[IBIS Ver]   4.0
[Comment Char] |_char
[File name]   pse84_bga220.ibs
[File Rev] 1.2
[Date] 10/27/2023
[Source] Infineon Technologies IBIS team
[Notes]
|Rev. 1.0 - Initial model 12/8/2021
|Rev. 1.1 - Update with RLC 8/17/2023
|Rev. 1.2 - Included pins for MIPI-DPHY DSI and USB 10/23/2023
|Supports 1.8 V IO Interface and 3.3 V RF Switch Control Interface.
|The temperature range is -40 to 125C.
|This model was syntax checked with Hyperlynx 4.2 visual IBIS
|editor and ibischk7_64 IBIS checker.
|There were 0 syntax errors.
[Disclaimer]   The model given below represents a 220-pin package.
[Copyright]   (C) COPYRIGHT 2023, Infineon Technologies AG.
[Component] PSOCE84
[Manufacturer] Infineon Technologies AG
| Package model BGA220 was extracted from simulation tool.
[Package]
|   typ   min   max
R_pkg   0.20796   0.07347   0.41266
L_pkg   2.2356n   0.87131n   4.135n
C_pkg   0.96052p   0.4552p   1.843p
[Pin]   Signal_name   model_name   R_pin   L_pin   C_pin
|A4   DSI_CLK_N_PAD   PAD   0.20054 2.35E-09 5.53E-13
|A5   DSI_CLK_P_PAD   PAD   0.16186 1.88E-09 4.79E-13
|B4   DSI_DATA0_N_PAD PAD   0.17864 1.75E-09 9.29E-13
|B3   DSI_DATA0_P_PAD PAD   0.2296  2.45E-09 8.54E-13
|A3   DSI_DATA1_N_PAD PAD   0.1872  2.24E-09 5.28E-13
|A2   DSI_DATA1_P_PAD PAD   0.23123 2.69E-09 6.88E-13
|J6   DSI_REXT_PAD   0.36792 3.61E-09 1.32E-12
K5   P0_0_PAD   Mpad 0.22656 2.30E-09 1.44E-12
C4   P0_1_PAD   Mpad 0.22018 2.42E-09 1.02E-12
B15   P10_0_PAD   1p8_ioi2c_wbso_h   0.21635 2.63E-09  6.76E-13
A13   P10_1_PAD   1p8_ioi2c_wbso_h   0.18836 2.05E-09  8.54E-13
C15   P10_2_PAD   1p8_ioi2c_wbso_h   0.2   2.52E-09  4.58E-13
A14   P10_3_PAD   1p8_ioi2c_wbso_h   0.2025  2.35E-09  7.28E-13
D14   P10_4_PAD   1p8_ioi2c_wbso_h   0.17929 2.22E-09  5.12E-13
B14   P10_5_PAD   1p8_ioi2c_wbso_h   0.18293 2.02E-09  8.32E-13
D15   P10_6_PAD   1p8_ioi2c_wbso_h   0.18633 2.26E-09  4.55E-13
C14   P10_7_PAD   1p8_ioi2c_wbso_h   0.16378 1.74E-09  8.10E-13
E14   P11_0_PAD   1p8_ovt_wbso_h  0.15753 1.75E-09   5.94E-13
E11   P11_1_PAD   1p8_ovt_wbso_h  0.13177 1.35E-09   1.04E-12
E15   P11_2_PAD   1p8_ovt_wbso_h  0.18244 2.22E-09   5.01E-13
E10   P11_3_PAD   1p8_ovt_wbso_h  0.16649 1.81E-09   9.34E-13
F14   P11_4_PAD   1p8_ovt_wbso_h  0.16571 1.97E-09   5.83E-13
F9   P11_5_PAD   1p8_ovt_wbso_h  0.16904 1.76E-09   1.03E-12
F13   P11_6_PAD   1p8_ovt_wbso_h  0.16654 1.72E-09   6.89E-13
F10   P11_7_PAD   1p8_ovt_wbso_h  0.14172 1.43E-09   9.11E-13
H5   P12_0_PAD   1p8_ioi2c_wbso_h   0.22824 2.31E-09   1.72E-12
D5   P12_1_PAD   1p8_ioi2c_wbso_h   0.3004  3.07E-09   1.08E-12
G5   P12_2_PAD   1p8_ioi2c_wbso_h   0.21503 2.22E-09   1.67E-12
E5   P12_3_PAD   1p8_ioi2c_wbso_h   0.3353  3.50E-09   1.22E-12
F4   P12_4_PAD   1p8_ioi2c_wbso_h   0.21904 2.27E-09   1.70E-12
F5   P12_5_PAD   1p8_ioi2c_wbso_h   0.35086 3.67E-09   1.26E-12
G8   P13_0_PAD   1p8_gpib_3swbso_h   0.17914 1.89E-09   1.14E-12
G9   P13_1_PAD   1p8_ioi2c_wbso_h   0.19087 1.96E-09   1.12E-12
G10   P13_2_PAD   1p8_ioi2c_wbso_h   0.16512 1.71E-09   1.02E-12
F15   P13_3_PAD   1p8_ioi2c_wbso_h   0.17042 1.84E-09   6.52E-13
G11   P13_4_PAD   1p8_ioi2c_wbso_h   0.11221 1.14E-09   9.78E-13
G14   P13_5_PAD   1p8_gpib_3swbso_h   0.17144 1.82E-09   5.45E-13
H11   P13_6_PAD   1p8_ioi2c_wbso_h   0.13435 1.39E-09   1.17E-12
H15   P13_7_PAD   1p8_ioi2c_wbso_h   0.1915  2.03E-09   5.03E-13
H10   P14_0_PAD   1p8_gpib_3swbso_h   0.16351 1.69E-09   1.38E-12
H13   P14_1_PAD   1p8_ioi2c_wbso_h   0.16226 1.59E-09   6.35E-13
H9   P14_2_PAD   1p8_ioi2c_wbso_h   0.18536 1.94E-09   1.41E-12
K15   P14_3_PAD   1p8_ioi2c_wbso_h   0.21748 2.73E-09   6.39E-13
J9   P14_4_PAD   1p8_ioi2c_wbso_h   0.17465 1.83E-09   1.32E-12
J15   P14_5_PAD   1p8_gpib_3swbso_h   0.17014 2.04E-09   5.24E-13
J10   P14_6_PAD   1p8_ioi2c_wbso_h   0.165   1.67E-09   1.02E-12
J14   P14_7_PAD   1p8_ioi2c_wbso_h   0.15607 1.59E-09   6.84E-13
L15   P15_0_PAD   1p8_ioi2c_wbso_h   0.17878 1.99E-09   6.08E-13
K13   P15_1_PAD   1p8_ioi2c_wbso_h   0.09136 9.76E-10   7.13E-13
M15   P15_2_PAD   1p8_ioi2c_wbso_h   0.21222 2.46E-09   6.00E-13
K9   P15_3_PAD   1p8_ioi2c_wbso_h   0.18524 1.95E-09   1.08E-12
N15   P15_4_PAD   1p8_ioi2c_wbso_h   0.21678 2.49E-09   7.87E-13
K10   P15_5_PAD   1p8_ioi2c_wbso_h   0.14996 1.62E-09   1.01E-12
P15   P15_6_PAD   1p8_ioi2c_wbso_h   0.26151 3.03E-09   7.66E-13
K11   P15_7_PAD   1p8_ioi2c_wbso_h   0.13152 1.43E-09   1.09E-12
M11   P16_0_PAD   3p3_gpio_wbso_v 0.15372 1.78E-09   8.07E-13
R13   P16_1_PAD   3p3_gpio_wbso_v 0.20685 2.25E-09   9.30E-13
N11   P16_2_PAD   3p3_gpio_wbso_v 0.18636 2.08E-09   8.28E-13
L11   P16_3_PAD   3p3_gpio_wbso_v 0.083686   9.67E-10   8.68E-13
P11   P16_4_PAD   3p3_gpio_wbso_v 0.21434 2.37E-09   8.02E-13
L10   P16_5_PAD   3p3_gpio_wbso_v 0.07347 8.73E-10   1.03E-12
R11   P16_6_PAD   3p3_gpio_wbso_v 0.22038 2.44E-09   7.88E-13
M10   P16_7_PAD   3p3_gpio_wbso_v 0.084206   9.06E-10   7.71E-13
M9   P17_0_PAD   3p3_gpio_wbso_v 0.15721 1.77E-09   8.06E-13
R9   P17_1_PAD   3p3_gpio_wbso_v 0.18702 1.89E-09   8.89E-13
R8   P17_2_PAD   3p3_gpio_wbso_v 0.22427 2.51E-09   8.66E-13
P9   P17_3_PAD   3p3_gpio_wbso_v 0.15414 1.64E-09   9.02E-13
P8   P17_4_PAD   3p3_gpio_wbso_v 0.19733 2.23E-09   8.36E-13
N9   P17_5_PAD   3p3_gpio_wbso_v 0.12454 1.32E-09   9.02E-13
N8   P17_6_PAD   3p3_gpio_wbso_v 0.18534 2.07E-09   8.23E-13
L9   P17_7_PAD   3p3_gpio_wbso_v 0.088819   9.54E-10   8.43E-13
G7   P18_0_PAD   1p8_gpib_3swbso_v   0.37774 3.96E-09   1.23E-12
H8   P18_1_PAD   1p8_gpib_3swbso_v   0.23204 2.41E-09   1.75E-12
B6   P19_0_PAD   1p8_gpib_3swbso_v   0.19164 2.27E-09   6.28E-13
F8   P19_1_PAD   1p8_gpib_3swbso_v   0.1648  1.77E-09   1.31E-12
K4   P2_0_PAD   Mpad   0.19132 1.92E-09   1.10E-12
P14   P20_0_PAD   1p8_ioi2c_wbso_h   0.22796 2.31E-09   1.03E-12
M12   P20_1_PAD   1p8_ioi2c_wbso_h   0.16258 1.85E-09   8.37E-13
R15   P20_2_PAD   1p8_ioi2c_wbso_h   0.24673 2.75E-09   9.68E-13
N12   P20_3_PAD   1p8_ioi2c_wbso_h   0.18993 2.15E-09   8.18E-13
R14   P20_4_PAD   1p8_ioi2c_wbso_h   0.24853 2.76E-09   9.15E-13
P12   P20_5_PAD   1p8_ioi2c_wbso_h   0.22155 2.48E-09   8.21E-13
P13   P20_6_PAD   1p8_ioi2c_wbso_h   0.17567 1.91E-09   9.23E-13
R12   P20_7_PAD   1p8_ioi2c_wbso_h   0.22524 2.55E-09   8.09E-13
J5   P21_0_PAD   1p8_ioi2c_wbso_h   0.23138 2.31E-09   1.55E-12
E4   P21_1_PAD   1p8_ioi2c_wbso_h   0.30704 3.17E-09   1.20E-12
K7   P21_2_PAD   1p8_ioi2c_wbso_h   0.27883 2.80E-09   1.64E-12
D4   P21_3_PAD   1p8_ioi2c_wbso_h   0.29341 3.06E-09   1.12E-12
K6   P21_4_PAD   1p8_ioi2c_wbso_h   0.24937 2.54E-09   1.56E-12
C5   P21_5_PAD   1p8_ioi2c_wbso_h   0.26732 2.84E-09   1.20E-12
L7   P21_6_PAD   1p8_ioi2c_wbso_h   0.28784 2.87E-09   1.52E-12
C3   P21_7_PAD   1p8_ioi2c_wbso_h   0.19023 2.11E-09   8.90E-13
M4   P3_0_PAD   1p8_ioi3c_3swbso_h   0.27521 2.73E-09   1.22E-12
L6   P3_1_PAD   1p8_ioi3c_3swbso_h   0.17463 1.82E-09   1.35E-12
J4   P5_0_PAD   Mpad   0.14852 1.49E-09   1.56E-12
M6   P6_0_PAD   1p8_ioi2c_wbso_h   0.15505 1.69E-09   8.65E-13
N6   P6_1_PAD   1p8_ioi2c_wbso_h   0.18486 2.04E-09   8.54E-13
P6   P6_2_PAD   1p8_ioi2c_wbso_h   0.21336 2.35E-09   7.99E-13
R6   P6_3_PAD   1p8_ioi2c_wbso_h   0.21761 2.42E-09   7.36E-13
R5   P6_4_PAD   1p8_ioi2c_wbso_h   0.22859 2.43E-09   1.00E-12
R2   P6_5_PAD   1p8_ioi2c_wbso_h   0.29623 3.21E-09   8.98E-13
P5   P6_6_PAD   1p8_ioi2c_wbso_h   0.20466 2.15E-09   1.01E-12
P2   P6_7_PAD   1p8_ioi2c_wbso_h   0.29712 2.98E-09   9.31E-13
P3   P7_0_PAD   1p8_ioi2c_wbso_h   0.27636 2.60E-09   1.03E-12
N5   P7_1_PAD   1p8_ioi2c_wbso_h   0.21064 2.19E-09   1.09E-12
R4   P7_2_PAD   1p8_ioi2c_wbso_h   0.30429 3.15E-09   1.15E-12
M5   P7_3_PAD   1p8_ioi2c_wbso_h   0.19338 2.05E-09   1.23E-12
P4   P7_4_PAD   1p8_ioi2c_wbso_h   0.2891  2.98E-09   1.13E-12
L4   P7_5_PAD   1p8_ioi2c_wbso_h   0.1324  1.41E-09   1.15E-12
N4   P7_6_PAD   1p8_ioi2c_wbso_h   0.29217 2.90E-09   1.15E-12
L5   P7_7_PAD   1p8_ioi2c_wbso_h   0.14611 1.56E-09   1.23E-12
H7   P8_0_PAD   1p8_ioi2c_wbso_h   0.39168 3.83E-09   1.31E-12
J8   P8_1_PAD   1p8_ioi2c_wbso_h   0.25811 2.68E-09   1.84E-12
J7   P8_2_PAD   1p8_ioi2c_wbso_h   0.41266 4.14E-09   1.43E-12
K8   P8_3_PAD   1p8_ioi2c_wbso_h   0.2804  2.80E-09   1.78E-12
F6   P8_4_PAD   1p8_ioi2c_wbso_h   0.27559 2.68E-09   1.04E-12
E7   P8_5_PAD   1p8_ioi2c_wbso_h   0.11114 1.15E-09   1.42E-12
G6   P8_6_PAD   1p8_ioi2c_wbso_h   0.29663 3.02E-09   1.19E-12
H6   P8_7_PAD   1p8_ioi2c_wbso_h   0.32423 3.31E-09   1.25E-12
L14   P9_0_PAD   1p8_ioi2c_wbso_h   0.11336 1.28E-09   6.46E-13
M13   P9_1_PAD   1p8_ioi2c_wbso_h   0.16723 1.93E-09   8.46E-13
M14   P9_2_PAD   1p8_ioi2c_wbso_h   0.15087 1.58E-09   8.83E-13
N13   P9_3_PAD   1p8_ioi2c_wbso_h   0.19382 2.18E-09   8.16E-13
L1   SMIF0_CLK_N_PAD Mpad_0   0.23622 2.67E-09   6.87E-13
M1   SMIF0_CLK_P_PAD Mpad_1   0.25153 2.76E-09   7.75E-13
N2   SMIF0_DATA0_PAD Mpad   0.29527 3.06E-09   1.12E-12
P1   SMIF0_DATA1_PAD Mpad   0.31791 3.40E-09   1.18E-12
N1   SMIF0_DATA2_PAD Mpad   0.31365 3.42E-09   9.23E-13
M2   SMIF0_DATA3_PAD Mpad   0.27296 2.87E-09   1.01E-12
L2   SMIF0_DATA4_PAD Mpad   0.25293 2.77E-09   9.73E-13
K2   SMIF0_DATA5_PAD Mpad   0.26485 2.86E-09   1.06E-12
K1   SMIF0_DATA6_PAD Mpad   0.26877 2.90E-09   8.60E-13
J2   SMIF0_DATA7_PAD Mpad   0.25994 2.81E-09   8.99E-13
J1   SMIF0_RWDS_PAD  Mpad   0.20375 2.49E-09   6.18E-13
F1   SMIF1_CLK_N_PAD Mpad_0   0.1842  2.21E-09   5.56E-13
E1   SMIF1_CLK_P_PAD Mpad_1   0.18934 2.20E-09   5.44E-13
C2   SMIF1_DATA0_PAD Mpad   0.18423 2.07E-09   7.99E-13
C1   SMIF1_DATA1_PAD Mpad   0.20375 2.29E-09   6.75E-13
D2   SMIF1_DATA2_PAD Mpad   0.18525 2.19E-09   6.35E-13
D1   SMIF1_DATA3_PAD Mpad   0.19093 2.32E-09   6.19E-13
F2   SMIF1_DATA4_PAD Mpad   0.19204 2.11E-09   7.77E-13
E2   SMIF1_DATA5_PAD Mpad   0.16192 1.78E-09   1.00E-12
G2   SMIF1_DATA6_PAD Mpad   0.1669  1.84E-09   7.17E-13
H2   SMIF1_DATA7_PAD Mpad   0.19427 2.18E-09   7.47E-13
H1   SMIF1_RWDS_PAD  Mpad   0.19851 2.24E-09   6.91E-13
|P7   USB_DM_PAD   PAD  0.20896 1.96E-09   8.83E-13
|N7   USB_DP_PAD   PAD  0.18134 1.68E-09   8.75E-13
H4   VCCD_0_PAD   POWER
F11   VCCD_1_PAD   POWER
E9   VCCD_2_PAD   POWER
M8   VCCD_3_PAD   POWER
B1   VCCD_4_PAD   POWER
B7   VCCD_ANA_PAD   POWER
B12   VCCI_SR_0_PAD   POWER
B13   VCCI_SR1P8_0_PAD   POWER
B9   VCCIRETLDO_PAD  POWER
C9   VCCRET_PAD   POWER
A8   VCCSRAM_PAD   POWER
F12   VCCSRAMI_0_PAD  POWER
K3   VCCSRAMI_1_PAD  POWER
M7   VDD33_USB_PAD   POWER
H14   VDDA_CTB_PAD   POWER
J12   VDDA_PAD   POWER
J11   VDDA_SAR_PAD   POWER
D10   VDDBAT_0_PAD   POWER
B11   VDDBAT_SR_PAD   POWER
G4   VDDD_DLL_PAD   POWER
A7   VDDD_PAD   POWER
B10   VDDD_SR_PAD   POWER
C12   VDDD_SR1P8_PAD  POWER
B8   VDDDLDO_PAD   POWER
R3   VDDIO_0_PAD   POWER
E6   VDDIO_1_PAD   POWER
R10   VDDIO_1P8_3P3_PAD   POWER
N14   VDDIO_2_PAD   POWER
E13   VDDIO_3_PAD   POWER
B2   VDDIO_4_PAD   POWER
G12   VDDIO_A_PAD   POWER
L12   VDDIO_A_Q_PAD   POWER
A6   VDDIO_CO_PAD   POWER
M3   VDDIO_SMIF0_0_PAD   POWER
J3   VDDIO_SMIF0_1_PAD   POWER
E3   VDDIO_SMIF1_0_PAD   POWER
G3   VDDIO_SMIF1_1_PAD   POWER
A12   VDDLX_SR_PAD   POWER
C13   VDDLX_SR1P8_PAD POWER
P10   VDDP_PAD   POWER
F7   VDDPUMP_RRAM_PAD   POWER
A11   VDDQ_0_PAD   POWER
A10   VDDQ_SR_PAD   POWER
A9   VDDQ_SR1P8_PAD  POWER
C6   VP_DSI_PAD   POWER
D6   VPH_P_DSI_PAD   POWER
C7   VPL_P_DSI_PAD   POWER
K14   VREF_PAD   POWER
C11   VSS_SR_PAD   GND
D12   VSS_SR1P8_PAD   GND
R7   VSS_USB_PAD   GND
G13   VSSA   GND
H12   VSSA   GND
J13   VSSA   GND
K12   VSSA   GND
L13   VSSA   GND
B5   VSSD   GND
D11   VSSD   GND
D13   VSSD   GND
D3   VSSD   GND
D7   VSSD   GND
E12   VSSD   GND
E8   VSSD   GND
F3   VSSD   GND
H3   VSSD   GND
L3   VSSD   GND
L8   VSSD   GND
N10   VSSD   GND
N3   VSSD   GND
C10   VSSQ_PAD   GND
C8   VSSQ_PAD   GND
D9   VSSQ_PAD   GND
D8   XRES_PAD   1p8_xres_3swbso 0.088991   9.56E-10   7.58E-13
[Diff_pin]   inv_pin   vdiff   tdelay_typ   tdelay_min   tdelay_max
E1   F1   0.2   -40.2244p   NA   NA
M1   L1   0.2   -40.2244p   NA   NA
|   MODEL SELECTOR
[Model Selector] 1p8_ioi2c_wbso_h
| Model Description
ioi2c_drive000_slew0   obuf mode with drive_sel=000 and slew_sel=0
ioi2c_drive000_slew1   obuf mode with drive_sel=000 and slew_sel=1
ioi2c_drive100_slew0   obuf mode with drive_sel=100 and slew_sel=0
ioi2c_drive100_slew1   obuf mode with drive_sel=100 and slew_sel=1
ioi2c_drive010_slew0   obuf mode with drive_sel=010 and slew_sel=0
ioi2c_drive010_slew1   obuf mode with drive_sel=010 and slew_sel=1
ioi2c_drive110_slew0   obuf mode with drive_sel=110 and slew_sel=0
ioi2c_drive110_slew1   obuf mode with drive_sel=110 and slew_sel=1
ioi2c_drive001_slew0   obuf mode with drive_sel=001 and slew_sel=0
ioi2c_drive001_slew1   obuf mode with drive_sel=001 and slew_sel=1
ioi2c_drive101_slew0   obuf mode with drive_sel=101 and slew_sel=0
ioi2c_drive101_slew1   obuf mode with drive_sel=101 and slew_sel=1
ioi2c_drive011_slew0   obuf mode with drive_sel=011 and slew_sel=0
ioi2c_drive011_slew1   obuf mode with drive_sel=011 and slew_sel=1
ioi2c_drive111_slew0   obuf mode with drive_sel=111 and slew_sel=0
ioi2c_drive111_slew1   obuf mode with drive_sel=111 and slew_sel=1
ioi2c_drive000_slow1   obuf mode with drive_sel=000 and slow=1
ioi2c_drive100_slow1   obuf mode with drive_sel=100 and slow=1
ioi2c_drive010_slow1   obuf mode with drive_sel=010 and slow=1
ioi2c_drive110_slow1   obuf mode with drive_sel=110 and slow=1
ioi2c_drive001_slow1   obuf mode with drive_sel=001 and slow=1
ioi2c_drive101_slow1   obuf mode with drive_sel=101 and slow=1
ioi2c_drive011_slow1   obuf mode with drive_sel=011 and slow=1
ioi2c_drive111_slow1   obuf mode with drive_sel=111 and slow=1
[Model Selector] 1p8_ioi3c_3swbso_h
| Model Description
ioi3c_drive000_slew0   obuf mode with drive_sel=000 and slew_sel=0
ioi3c_drive000_slew1   obuf mode with drive_sel=000 and slew_sel=1
ioi3c_drive100_slew0   obuf mode with drive_sel=100 and slew_sel=0
ioi3c_drive100_slew1   obuf mode with drive_sel=100 and slew_sel=1
ioi3c_drive010_slew0   obuf mode with drive_sel=010 and slew_sel=0
ioi3c_drive010_slew1   obuf mode with drive_sel=010 and slew_sel=1
ioi3c_drive110_slew0   obuf mode with drive_sel=110 and slew_sel=0
ioi3c_drive110_slew1   obuf mode with drive_sel=110 and slew_sel=1
ioi3c_drive001_slew0   obuf mode with drive_sel=001 and slew_sel=0
ioi3c_drive001_slew1   obuf mode with drive_sel=001 and slew_sel=1
ioi3c_drive101_slew0   obuf mode with drive_sel=101 and slew_sel=0
ioi3c_drive101_slew1   obuf mode with drive_sel=101 and slew_sel=1
ioi3c_drive011_slew0   obuf mode with drive_sel=011 and slew_sel=0
ioi3c_drive011_slew1   obuf mode with drive_sel=011 and slew_sel=1
ioi3c_drive111_slew0   obuf mode with drive_sel=111 and slew_sel=0
ioi3c_drive111_slew1   obuf mode with drive_sel=111 and slew_sel=1
ioi3c_drive000_slow1   obuf mode with drive_sel=000 and slow=1
ioi3c_drive100_slow1   obuf mode with drive_sel=100 and slow=1
ioi3c_drive010_slow1   obuf mode with drive_sel=010 and slow=1
ioi3c_drive110_slow1   obuf mode with drive_sel=110 and slow=1
ioi3c_drive001_slow1   obuf mode with drive_sel=001 and slow=1
ioi3c_drive101_slow1   obuf mode with drive_sel=101 and slow=1
ioi3c_drive011_slow1   obuf mode with drive_sel=011 and slow=1
ioi3c_drive111_slow1   obuf mode with drive_sel=111 and slow=1
[Model Selector] 1p8_ovt_wbso_h
| Model Description
ovt_000_slew0   obuf mode with drive_sel=000 and slew_sel=0
ovt_000_slew1   obuf mode with drive_sel=000 and slew_sel=1
ovt_100_slew0   obuf mode with drive_sel=100 and slew_sel=0
ovt_100_slew1   obuf mode with drive_sel=100 and slew_sel=1
ovt_010_slew0   obuf mode with drive_sel=010 and slew_sel=0
ovt_010_slew1   obuf mode with drive_sel=010 and slew_sel=1
ovt_110_slew0   obuf mode with drive_sel=110 and slew_sel=0
ovt_110_slew1   obuf mode with drive_sel=110 and slew_sel=1
ovt_001_slew0   obuf mode with drive_sel=001 and slew_sel=0
ovt_001_slew1   obuf mode with drive_sel=001 and slew_sel=1
ovt_101_slew0   obuf mode with drive_sel=101 and slew_sel=0
ovt_101_slew1   obuf mode with drive_sel=101 and slew_sel=1
ovt_011_slew0   obuf mode with drive_sel=011 and slew_sel=0
ovt_011_slew1   obuf mode with drive_sel=011 and slew_sel=1
ovt_111_slew0   obuf mode with drive_sel=111 and slew_sel=0
ovt_111_slew1   obuf mode with drive_sel=111 and slew_sel=1
ovt_000_slow1   obuf mode with drive_sel=000 and slow=1
ovt_100_slow1   obuf mode with drive_sel=100 and slow=1
ovt_010_slow1   obuf mode with drive_sel=010 and slow=1
ovt_110_slow1   obuf mode with drive_sel=110 and slow=1
ovt_001_slow1   obuf mode with drive_sel=001 and slow=1
ovt_101_slow1   obuf mode with drive_sel=101 and slow=1
ovt_011_slow1   obuf mode with drive_sel=011 and slow=1
ovt_111_slow1   obuf mode with drive_sel=111 and slow=1
[Model Selector] 3p3_gpio_wbso_v
| Model Description
gpio_000_slew0_slow0   obuf mode with drive_sel=000 and slew_sel=0
gpio_000_slew1_slow0   obuf mode with drive_sel=000 and slew_sel=1
gpio_100_slew0_slow0   obuf mode with drive_sel=100 and slew_sel=0
gpio_100_slew1_slow0   obuf mode with drive_sel=100 and slew_sel=1
gpio_010_slew0_slow0   obuf mode with drive_sel=010 and slew_sel=0
gpio_010_slew1_slow0   obuf mode with drive_sel=010 and slew_sel=1
gpio_110_slew0_slow0   obuf mode with drive_sel=110 and slew_sel=0
gpio_110_slew1_slow0   obuf mode with drive_sel=110 and slew_sel=1
gpio_001_slew0_slow0   obuf mode with drive_sel=001 and slew_sel=0
gpio_001_slew1_slow0   obuf mode with drive_sel=001 and slew_sel=1
gpio_101_slew0_slow0   obuf mode with drive_sel=101 and slew_sel=0
gpio_101_slew1_slow0   obuf mode with drive_sel=101 and slew_sel=1
gpio_011_slew0_slow0   obuf mode with drive_sel=011 and slew_sel=0
gpio_011_slew1_slow0   obuf mode with drive_sel=011 and slew_sel=1
gpio_111_slew0_slow0   obuf mode with drive_sel=111 and slew_sel=0
gpio_111_slew1_slow0   obuf mode with drive_sel=111 and slew_sel=1
gpio_000_slew0_slow1   obuf mode with drive_sel=000 for slow=1 and slew=0
gpio_000_slew1_slow1   obuf mode with drive_sel=000 for slow=1 and slew=1
gpio_100_slew0_slow1   obuf mode with drive_sel=100 for slow=1 and slew=0
gpio_100_slew1_slow1   obuf mode with drive_sel=100 for slow=1 and slew=1
gpio_010_slew0_slow1   obuf mode with drive_sel=010 for slow=1 and slew=0
gpio_010_slew1_slow1   obuf mode with drive_sel=010 for slow=1 and slew=1
gpio_110_slew0_slow1   obuf mode with drive_sel=110 for slow=1 and slew=0
gpio_110_slew1_slow1   obuf mode with drive_sel=110 for slow=1 and slew=1
gpio_001_slew0_slow1   obuf mode with drive_sel=001 for slow=1 and slew=0
gpio_001_slew1_slow1   obuf mode with drive_sel=001 for slow=1 and slew=1
gpio_101_slew0_slow1   obuf mode with drive_sel=101 for slow=1 and slew=0
gpio_101_slew1_slow1   obuf mode with drive_sel=101 for slow=1 and slew=1
gpio_011_slew0_slow1   obuf mode with drive_sel=011 for slow=1 and slew=0
gpio_011_slew1_slow1   obuf mode with drive_sel=011 for slow=1 and slew=1
gpio_111_slew0_slow1   obuf mode with drive_sel=111 for slow=1 and slew=0
gpio_111_slew1_slow1   obuf mode with drive_sel=111 for slow=1 and slew=1
| pad
[Model Selector] Mpad
| Model Description
hsio_drive000_slew0  obuf mode with drive_sel=000 and slew_sel=0
hsio_drive000_slew1  obuf mode with drive_sel=000 and slew_sel=1
hsio_drive001_slew0  obuf mode with drive_sel=001 and slew_sel=0
hsio_drive001_slew1  obuf mode with drive_sel=001 and slew_sel=1
hsio_drive010_slew0  obuf mode with drive_sel=010 and slew_sel=0
hsio_drive010_slew1  obuf mode with drive_sel=010 and slew_sel=1
hsio_drive011_slew0  obuf mode with drive_sel=011 and slew_sel=0
hsio_drive011_slew1  obuf mode with drive_sel=011 and slew_sel=1
hsio_drive100_slew0  obuf mode with drive_sel=100 and slew_sel=0
hsio_drive100_slew1  obuf mode with drive_sel=100 and slew_sel=1
hsio_drive101_slew0  obuf mode with drive_sel=101 and slew_sel=0
hsio_drive101_slew1  obuf mode with drive_sel=101 and slew_sel=1
hsio_drive110_slew0  obuf mode with drive_sel=110 and slew_sel=0
hsio_drive110_slew1  obuf mode with drive_sel=110 and slew_sel=1
hsio_drive111_slew0  obuf mode with drive_sel=111 and slew_sel=0
hsio_drive111_slew1  obuf mode with drive_sel=111 and slew_sel=1
[Model Selector] Mpad_0
| Model Description
p0_drive000_slew0  obuf mode with drive_sel=000 and slew_sel=0
p0_drive000_slew1  obuf mode with drive_sel=000 and slew_sel=1
p0_drive001_slew0  obuf mode with drive_sel=001 and slew_sel=0
p0_drive001_slew1  obuf mode with drive_sel=001 and slew_sel=1
p0_drive010_slew0  obuf mode with drive_sel=010 and slew_sel=0
p0_drive010_slew1  obuf mode with drive_sel=010 and slew_sel=1
p0_drive011_slew0  obuf mode with drive_sel=011 and slew_sel=0
p0_drive011_slew1  obuf mode with drive_sel=011 and slew_sel=1
p0_drive100_slew0  obuf mode with drive_sel=100 and slew_sel=0
p0_drive100_slew1  obuf mode with drive_sel=100 and slew_sel=1
p0_drive101_slew0  obuf mode with drive_sel=101 and slew_sel=0
p0_drive101_slew1  obuf mode with drive_sel=101 and slew_sel=1
p0_drive110_slew0  obuf mode with drive_sel=110 and slew_sel=0
p0_drive110_slew1  obuf mode with drive_sel=110 and slew_sel=1
p0_drive111_slew0  obuf mode with drive_sel=111 and slew_sel=0
p0_drive111_slew1  obuf mode with drive_sel=111 and slew_sel=1
[Model Selector] Mpad_1
| Model Description
p1_drive000_slew0  obuf mode with drive_sel=000 and slew_sel=0
p1_drive000_slew1  obuf mode with drive_sel=000 and slew_sel=1
p1_drive001_slew0  obuf mode with drive_sel=001 and slew_sel=0
p1_drive001_slew1  obuf mode with drive_sel=001 and slew_sel=1
p1_drive010_slew0  obuf mode with drive_sel=010 and slew_sel=0
p1_drive010_slew1  obuf mode with drive_sel=010 and slew_sel=1
p1_drive011_slew0  obuf mode with drive_sel=011 and slew_sel=0
p1_drive011_slew1  obuf mode with drive_sel=011 and slew_sel=1
p1_drive100_slew0  obuf mode with drive_sel=100 and slew_sel=0
p1_drive100_slew1  obuf mode with drive_sel=100 and slew_sel=1
p1_drive101_slew0  obuf mode with drive_sel=101 and slew_sel=0
p1_drive101_slew1  obuf mode with drive_sel=101 and slew_sel=1
p1_drive110_slew0  obuf mode with drive_sel=110 and slew_sel=0
p1_drive110_slew1  obuf mode with drive_sel=110 and slew_sel=1
p1_drive111_slew0  obuf mode with drive_sel=111 and slew_sel=0
p1_drive111_slew1  obuf mode with drive_sel=111 and slew_sel=1
| Models and submodels in the file (155): 1p8_gpib_3swbso_h (Input), 1p8_gpib_3swbso_v (Input), ioi2c_drive000_slew0 (I/O), ioi2c_drive000_slew1 (I/O), ioi2c_drive100_slew0 (I/O), ioi2c_drive100_slew1 (I/O), ioi2c_drive010_slew0 (I/O), ioi2c_drive010_slew1 (I/O), ioi2c_drive110_slew0 (I/O), ioi2c_drive110_slew1 (I/O), ioi2c_drive001_slew0 (I/O), ioi2c_drive001_slew1 (I/O), ioi2c_drive101_slew0 (I/O), ioi2c_drive101_slew1 (I/O), ioi2c_drive011_slew0 (I/O), ioi2c_drive011_slew1 (I/O), ioi2c_drive111_slew0 (I/O), ioi2c_drive111_slew1 (I/O), ioi2c_drive000_slow1 (I/O), ioi2c_drive100_slow1 (I/O), ioi2c_drive010_slow1 (I/O), ioi2c_drive110_slow1 (I/O), ioi2c_drive001_slow1 (I/O), ioi2c_drive101_slow1 (I/O), ioi2c_drive011_slow1 (I/O), ioi2c_drive111_slow1 (I/O), ioi3c_drive000_slew0 (I/O), ioi3c_drive000_slew1 (I/O), ioi3c_drive100_slew0 (I/O), ioi3c_drive100_slew1 (I/O), ioi3c_drive010_slew0 (I/O), ioi3c_drive010_slew1 (I/O), ioi3c_drive110_slew0 (I/O), ioi3c_drive110_slew1 (I/O), ioi3c_drive001_slew0 (I/O), ioi3c_drive001_slew1 (I/O), ioi3c_drive101_slew0 (I/O), ioi3c_drive101_slew1 (I/O), ioi3c_drive011_slew0 (I/O), ioi3c_drive011_slew1 (I/O), ioi3c_drive111_slew0 (I/O), ioi3c_drive111_slew1 (I/O), ioi3c_drive000_slow1 (I/O), ioi3c_drive100_slow1 (I/O), ioi3c_drive010_slow1 (I/O), ioi3c_drive110_slow1 (I/O), ioi3c_drive001_slow1 (I/O), ioi3c_drive101_slow1 (I/O), ioi3c_drive011_slow1 (I/O), ioi3c_drive111_slow1 (I/O), ovt_000_slew0 (I/O), ovt_000_slew1 (I/O), ovt_100_slew0 (I/O), ovt_100_slew1 (I/O), ovt_010_slew0 (I/O), ovt_010_slew1 (I/O), ovt_110_slew0 (I/O), ovt_110_slew1 (I/O), ovt_001_slew0 (I/O), ovt_001_slew1 (I/O), ovt_101_slew0 (I/O), ovt_101_slew1 (I/O), ovt_011_slew0 (I/O), ovt_011_slew1 (I/O), ovt_111_slew0 (I/O), ovt_111_slew1 (I/O), ovt_000_slow1 (I/O), ovt_100_slow1 (I/O), ovt_010_slow1 (I/O), ovt_110_slow1 (I/O), ovt_001_slow1 (I/O), ovt_101_slow1 (I/O), ovt_011_slow1 (I/O), ovt_111_slow1 (I/O), 1p8_xres_3swbso (Input), gpio_000_slew0_slow0 (I/O), gpio_000_slew1_slow0 (I/O), gpio_100_slew0_slow0 (I/O), gpio_100_slew1_slow0 (I/O), gpio_010_slew0_slow0 (I/O)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
